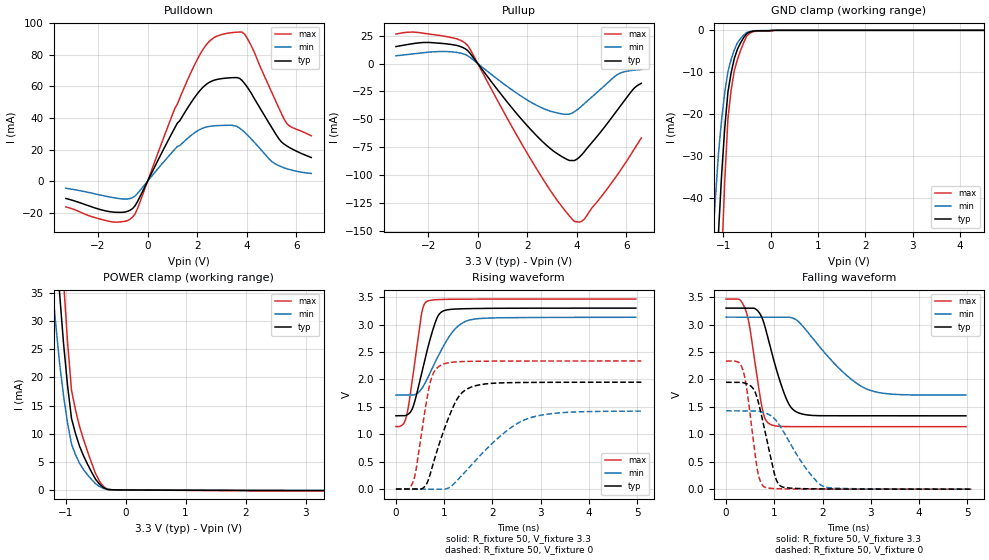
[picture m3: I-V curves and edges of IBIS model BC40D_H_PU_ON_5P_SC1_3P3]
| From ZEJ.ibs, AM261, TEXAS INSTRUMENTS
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[Model]   BC40D_H_PU_ON_5P_SC1_3P3
Model_type   I/O
Polarity   Non-Inverting
Enable   Active-Low
Vinl =  0.8V
Vinh =  2V
Cref =  15pF
Rref =  100.0000M
Vref =  0V
Vmeas =  1.65
C_comp   2.157014p   1.964007p   2.198404p
|[Input load] weak_pu_on
|[Output drive] slow
|[supplytol] 5
|[temp] ind
[Model Spec]
Vinl   0.8V   0.8V   0.8V
Vinh   2V   2V   2V
[Temperature Range]   25   125   -40
[Voltage Range]   3.3   3.135   3.465
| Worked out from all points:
|   slope of the pulldown table from 0 to 0.495 V, typ, clamps not added: 31.8 ohm
|   slope of the pullup table from 0 to 0.495 V, typ, clamps not added: 33.8 ohm
|   GND clamp passes 1 mA (typ) near -0.52 V on its own axis
|   POWER clamp passes 1 mA (typ) near -0.43 V on its own axis
|   rising waveform, R_fixture 50, V_fixture 3.3: 20-80 % time 338ps typ, 517ps min, 220ps max; typ from 1.34 V to 3.3 V
|   rising waveform, R_fixture 50, V_fixture 0: 20-80 % time 469ps typ, 1.01ns min, 253ps max; typ from 0.003 V to 1.95 V
|   falling waveform, R_fixture 50, V_fixture 3.3: 20-80 % time 388ps typ, 896ps min, 241ps max; typ from 3.3 V to 1.34 V
|   falling waveform, R_fixture 50, V_fixture 0: 20-80 % time 295ps typ, 612ps min, 205ps max; typ from 1.95 V to 0.002 V
| Nom Voltages:
|   VDD=1.1, VDDS=3.3, VDDS18=1.8, ESD_BIASFET=0, VSS=0, VSSS=0
| Min Voltages:
|   VDD=1.045, VDDS=3.135, VDDS18=1.71, ESD_BIASFET=0, VSS=0, VSSS=0
| Max Voltages:
|   VDD=1.16, VDDS=3.465, VDDS18=1.89, ESD_BIASFET=0, VSS=0, VSSS=0
[POWER_clamp]
|   voltage   I(typ)   I(min)   I(max)
-3.3V     446.9mA    437.1mA    604mA
-1.233V   56.55mA    37.5mA     80.28mA
-1.167V   45.63mA    29.89mA    65.07mA
-1.1V     35.1mA     22.65mA    50.26mA
-1.033V   26.08mA    16.75mA    37.2mA
-966.7mV  18.62mA    11.92mA    26.34mA
-900mV    12.7mA     8.144mA    17.7mA
-833.3mV  10mA       6.261mA    14.22mA
-766.7mV  7.795mA    4.75mA     11.31mA
-566.7mV  3.199mA    1.871mA    4.824mA
-366.7mV  433.5uA    268.9uA    617.1uA
3.3V      -100.3uA   -54.66uA   -173.1uA
[Pulldown]
|   voltage   I(typ)   I(min)   I(max)
-3.3V     -10.93mA   -4.474mA   -16.27mA
-1.4V     -19.53mA   -10.38mA   -25.83mA
-600mV    -17.23mA   -10.34mA   -22.61mA
1.2V      36.72mA    21.93mA    48.77mA
1.9V      53.02mA    30.66mA    73.76mA
2.4V      61.61mA    34.34mA    86.89mA
3V        64.86mA    35.24mA    92.76mA
3.6V      65.51mA    34.65mA    94.24mA
3.9V      62.01mA    31.1mA     93.16mA
5V        34.1mA     12.57mA    56.41mA
5.6V      22.42mA    7.958mA    36.79mA
6.6V      14.97mA    4.886mA    28.74mA
[Pullup]
|   voltage   I(typ)   I(min)   I(max)
-3.3V     15.12mA    6.907mA    26.36mA
-1.9V     18.73mA    10.27mA    26.12mA
-900mV    16.4mA     10.09mA    22.38mA
-400mV    11.39mA    6.888mA    15.9mA
1.3V      -37.44mA   -22.28mA   -53.31mA
2.4V      -65.08mA   -37.64mA   -95.03mA
3.3V      -81.9mA    -44.62mA   -125mA
3.9V      -86.71mA   -43.1mA    -141mA
4.3V      -78.82mA   -35.86mA   -139.1mA
5.6V      -42.54mA   -10.35mA   -100.4mA
6.3V      -22.29mA   -5.95mA    -77mA
6.6V      -17.71mA   -5.359mA   -66.44mA
[GND_clamp]
|   voltage   I(typ)   I(min)   I(max)
-3.3V     -787.2mA   -627.7mA   -1.235A
-1.233V   -85.67mA   -52.14mA   -138.8mA
-1.167V   -66.48mA   -40.37mA   -107.8mA
-1.1V     -48.26mA   -29.38mA   -78.01mA
-1.033V   -34.3mA    -21.2mA    -54.61mA
-966.7mV  -23.1mA    -14.68mA   -35.59mA
-900mV    -14.66mA   -9.807mA   -20.94mA
-833.3mV  -10.12mA   -6.96mA    -14.29mA
-700mV    -4.501mA   -2.971mA   -6.963mA
-500mV    -717.7uA   -493.4uA   -1.262mA
100mV     0A         0A         0A
6.6V      0A         0A         0A
[Ramp]
| variable   typ   min   max
dV/dt_f  1.1794644/0.38910928n 0.85575877/0.90218247n  1.3971095/0.24122653n
dV/dt_r  1.1737479/0.47008001n 0.86220396/1.0196273n   1.405963/0.2540815n
R_load = 50
[Rising Waveform]
R_fixture = 50
V_fixture = 3.3
V_fixture_min = 3.135
V_fixture_max = 3.465
|   time   V(typ)   V(min)   V(max)
0s        1.338V     1.715V     1.141V
142.6ps   1.338V     1.715V     1.178V
221.5ps   1.35V      1.715V     1.338V
358.9ps   1.509V     1.717V     2.112V
529.6ps   2.1V       1.825V     3.185V
642.5ps   2.512V     2V         3.421V
912.9ps   3.206V     2.488V     3.457V
1.205ns   3.282V     2.899V     3.462V
1.502ns   3.29V      3.076V     3.463V
4.974ns   3.3V       3.133V     3.465V
[Rising Waveform]
R_fixture = 50
V_fixture = 0
V_fixture_min = 0
V_fixture_max = 0
|   time   V(typ)   V(min)   V(max)
0s        2.605mV    0V         2.975mV
263.8ps   2.605mV    0V         2.975mV
361.7ps   2.605mV    0V         148.7mV
578.1ps   31.31mV    0V         1.3V
704.2ps   255.5mV    0V         1.921V
935.1ps   923.9mV    0V         2.261V
1.278ns   1.657V     165.3mV    2.322V
1.632ns   1.881V     506.4mV    2.331V
2.804ns   1.946V     1.306V     2.336V
5.089ns   1.949V     1.423V     2.336V
[Falling Waveform]
R_fixture = 50
V_fixture = 3.3
V_fixture_min = 3.135
V_fixture_max = 3.465
|   time   V(typ)   V(min)   V(max)
0s        3.299V     3.135V     3.464V
275.8ps   3.299V     3.135V     3.457V
414.1ps   3.299V     3.135V     3.243V
751.9ps   3.111V     3.135V     1.465V
907.2ps   2.625V     3.135V     1.187V
1.258ns   1.631V     3.135V     1.142V
1.518ns   1.387V     3.04V      1.141V
2.338ns   1.339V     2.208V     1.14V
2.91ns    1.339V     1.828V     1.14V
4.974ns   1.338V     1.718V     1.14V
[Falling Waveform]
R_fixture = 50
V_fixture = 0
V_fixture_min = 0
V_fixture_max = 0
|   time   V(typ)   V(min)   V(max)
0s        1.948V     1.428V     2.335V
356.3ps   1.941V     1.428V     2.151V
438.7ps   1.918V     1.428V     1.775V
650.5ps   1.648V     1.425V     347mV
797.7ps   1.098V     1.394V     39.64mV
1.022ns   221.5mV    1.268V     10.92mV
1.177ns   39.71mV    1.07V      6.907mV
1.666ns   9.651mV    369.6mV    3.316mV
2.042ns   6.092mV    46.11mV    3.012mV
5.089ns   2.107mV    3.418mV    2.776mV
